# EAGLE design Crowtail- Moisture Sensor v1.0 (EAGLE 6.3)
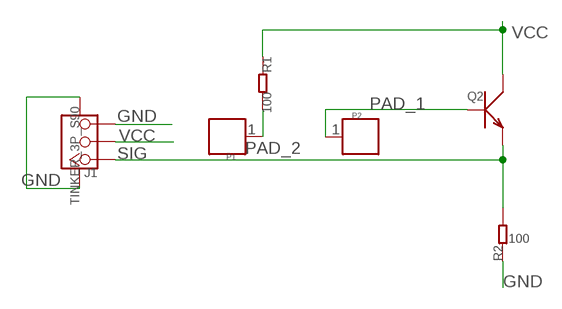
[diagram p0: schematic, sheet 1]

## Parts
J1  TINKER_3P_S90  [TINKER_3P_S90]
P1  PAD.03  [1P-SMD-0.76X0.76]
P2  PAD.03  [1P-SMD-0.76X0.76]
Q2  TRANSISTOR-NPN-SOT23''  [SOT23]
R1  100  R-0603  [0603]
R2  100  R-0603  [0603]

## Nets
GND: J1.3 J1.SS1 J1.SS2 R2.1
PAD_1: P2.1 Q2.1(B)
PAD_2: P1.1 R1.2
SIG: J1.1 Q2.2(E) R2.2
VCC: J1.2 Q2.3(C) R1.1

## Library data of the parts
J1 = Connector:TINKER_3P_S90
P1 P2 = Discrete:PAD
Q2 = Discrete:TRANSISTOR-NPN*: NPN audion
R1 R2 = Discrete:R*

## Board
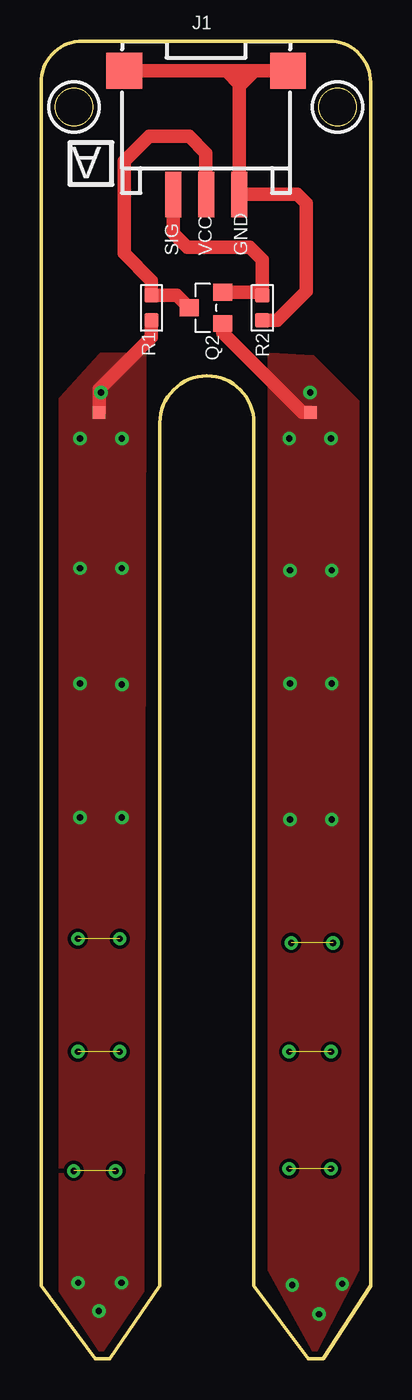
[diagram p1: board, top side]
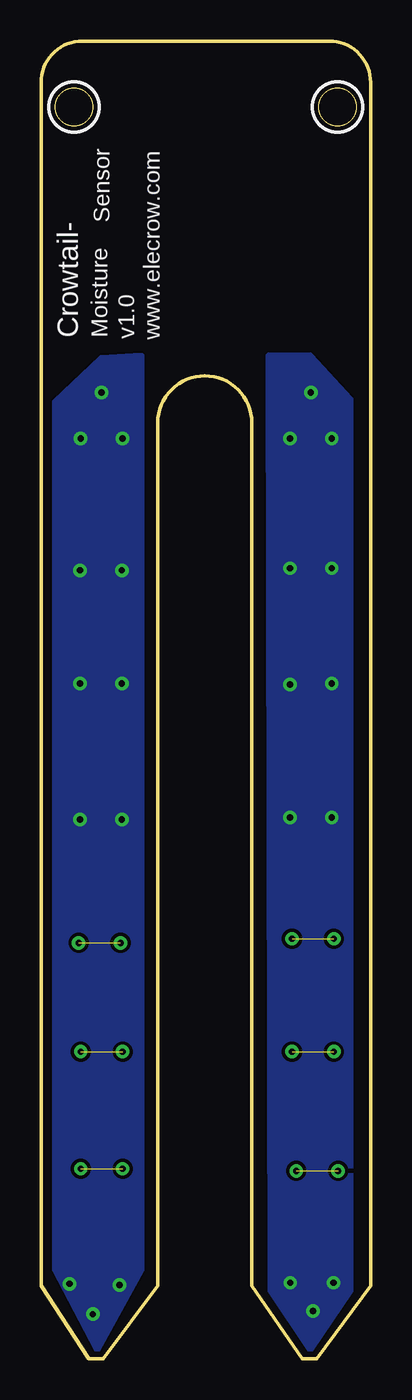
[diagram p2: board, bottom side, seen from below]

Size 20 x 80 mm. Coordinates in mm from the lower left corner, seen from the top.
Outline: 0,4.44 0,77.5 arc-90 2.5,80 17.5,80 arc-90 20,77.5 20,4.44 17.11,0 16.22,0 12.92,4.44 12.92,56.83 arc180 7.21,56.83 7.21,4.44 4.16,0 3.27,0 0,4.44
Outline: circle at 2,76 radius 1.14
Outline: circle at 18,76 radius 1.14
Copper layers (1*16): Top 0.035mm / dielectric 1.5mm / Bottom 0.035mm
Design rules "default *": minimum track width 10mil, minimum drill 12mil, track to track 8mil, track to pad 8mil, pad to pad 8mil, via to via 8mil, smd to smd 8mil, copper to edge 0mil, drill to drill 8mil, minimum pad ring 10mil, minimum via ring 8mil, stop-mask expansion 4mil, vias tented up to drill 25mil, thermal gap 10mil
tRestrict: area 0.5,74.5 to 3.5,77.5; area 16.5,74.5 to 19.5,77.5
bRestrict: area 0.5,74.5 to 3.5,77.5; area 16.5,74.5 to 19.5,77.5

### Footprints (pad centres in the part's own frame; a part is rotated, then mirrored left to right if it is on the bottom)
TINKER_3P_S90 = smd 0.965 x 2.74: 1 -1.984,-4.545; 2 0.016,-4.545; 3 2.016,-4.545 | smd 2.159 x 2.184: SS1 -4.958,2.955; SS2 4.99,2.955
1P-SMD-0.76X0.76 = smd 0.762 x 0.762: 1 0,0
SOT23 = smd 1.016 x 1.143: 1 -0.95,-1.016; 2 0.95,-1.016; 3 0,1.016
0603 = smd 0.889 x 0.889: 1 -0.762,0; 2 0.762,0

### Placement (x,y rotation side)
J1  10,75.24 0 top
P1  3.52,57.46 0 top
P2  16.35,57.46 0 top
Q2  10,63.81 90 top
R1  6.7,63.81 270 top
R2  13.43,63.81 90 top

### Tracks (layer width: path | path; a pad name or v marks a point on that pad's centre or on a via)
GND
  Top 0.813: R2.1 14.32,63.05 16.1,64.83 16.1,70.16 15.56,70.69 J1.3 12.03,70.71 12.03,77.27 12.96,78.19 J1.SS2 J1.SS1
N$1
  Top 0.813: 11.27,78.16 12.03,77.4
PAD_1  (via drill 0.38 pad 0.81)
  Top 0.813: P2.1 15.84,57.46 11.02,62.29 Q2.1
  other vias: 15.25,4.49 16.87,2.71 18.28,4.55 15.06,55.87 15.1,47.87 15.1,41 15.1,32.75 17.64,32.75 17.64,41 17.64,47.87 17.6,55.87 16.33,58.67
  pour Top (no thermals): 13.94,5.4 13.94,60.89 16.48,60.76 19.14,58.09 19.14,5.4 16.6,0.56
  pour Bottom (no thermals): 13.94,5.4 13.94,60.89 16.35,60.76 19.14,58.09 19.14,5.4 16.6,0.56
PAD_2  (via drill 0.38 pad 0.81)
  Top 0.813: 3.52,58.35 P1.1 3.52,58.86 6.7,62.03 R1.2
  other vias: 2.25,4.62 4.88,4.62 2.36,32.87 3.5,2.9 3.63,58.67 4.9,32.87 4.9,40.94 2.36,41 4.9,48 2.36,48 4.9,55.87 2.36,55.87
  pour Top (no thermals): 1.24,58.27 3.65,60.89 6.19,60.89 6.06,4.12 3.65,0.56 1.24,4.12
  pour Bottom (no thermals): 1.24,58.27 3.65,60.89 6.19,60.89 6.06,4.12 3.65,0.56 1.24,4.12
PAD_3  (via drill 0.38 pad 0.81)  (1 unrouted)
  other vias: 2.23,25.51 4.77,25.51
PAD_4  (via drill 0.38 pad 0.81)  (1 unrouted)
  other vias: 2.23,18.65 4.77,18.65
PAD_5  (via drill 0.38 pad 0.81)  (1 unrouted)
  other vias: 1.98,11.41 4.52,11.41
PAD_6  (via drill 0.38 pad 0.81)  (1 unrouted)
  other vias: 15.18,25.25 17.72,25.25
PAD_7  (via drill 0.38 pad 0.81)  (1 unrouted)
  other vias: 15.06,18.65 17.6,18.65
PAD_8  (via drill 0.38 pad 0.81)  (1 unrouted)
  other vias: 15.06,11.54 17.6,11.54
SIG
  Top 0.813: 13.43,65.08 13.43,66.73 12.67,67.49 8.86,67.49 8.02,68.33 J1.1 | 13.43,65.08 R2.2 | Q2.2 13.11,64.76 13.43,65.08
VCC
  Top 0.813: J1.2 10,70.68 10,73.21 8.98,74.22 6.57,74.22 5.05,72.7 5.05,67.11 6.7,65.46 R1.1 8.22,64.57 Q2.3

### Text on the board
tPlace: A | SIG | VCC | GND
bPlace: Sensor | www.elecrow.com | v1.0 | Moisture | Crowtail-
